| TEXAS INSTRUMENTS INCORPORATED
| Standard Linear and Logic Group
| IBIS Model of SN74LVC1G17
| SINGLE SCHMITT-TRIGGER BUFFER
| This file contains package information for the following:
|  SON 6-pin (DSF) package as [Component] LVC1G17_DSF
|  SOT 5-pin (DCK) package as [Component] LVC1G17_DCK
|  SOT 5-pin (DBV) package as [Component] LVC1G17_DBV
|  NanoStar WCSP 5-pin (YEA) package as [Component] LVC1G17_YEA
|  NanoFree WCSP 5-pin (YZA) package as [Component] LVC1G17_YZA
|  NanoStar WCSP 5-pin (YEP) package as [Component] LVC1G17_YEP
|  NanoFree WCSP 5-pin (YZP) package as [Component] LVC1G17_YZP
|  DSBGA 4-pin (YZV) package as [Component] LVC1G17_YZV
| This device can be powered at the following Vccs:
|  1.8 volt Vcc
|  2.5 volt Vcc
|  3.3 volt Vcc
|  5 volt Vcc
| This file provides unique models under the [Model Selector] for each Vcc.
| For operation at a specific Vcc, select the appropriate model after each
| [Model Selector] keyword.
[IBIS Ver]   3.2
[Comment char]  |_char
[File Name]   sn74lvc1g17.ibs
[File Rev]   1.4 | d_die
[Date]   03/06/2014
[Source]
| Texas Instruments Incorporated.
| Analog-eLab Design Center, HPA
| 12500 TI Blvd
| Dallas, TX -75243
[Notes]   Revision History:
| The following is an IBIS list for the LVC1G17.
| Please contact sllibis@ti.com with questions and
| comments concerning SLL IBIS models.
| - FILE REV HISTORY
| - 1.3 YZV package added on 12/21/05
| - Due to the fact that the Device is 5.5-V Input tolarent,
|   the pulldown model has some Non-Monotonic Warnings.
| - Power clamp data deleted as there is no power-clamp diode.
| - 1.4 DSF package added 03/06/2014.
[Disclaimer]
| Property of Texas Instruments Incorporated.  Unauthorized
| reproduction and/or distribution is strictly prohibited.
| This product is protected under copyright law.
| Created  2002, (C) Copyright  2002, Texas Instruments
| Incorporated, All Rights Reserved
| UNLESS THERE IS A SIGNED, WRITTEN AGREEMENT TO THE
| CONTRARY, TEXAS INSTRUMENTS (TI) IS PROVIDING THE IBIS
| MODELS  AND WITHOUT ANY WARRANTY, EXPRESSED OR
| IMPLIED.  TI assumes no liability for:
|  1) the accuracy of the IBIS models provided to your
|   company;
|  2) the proper functioning of these IBIS Models in your
|   design or for any resulting applications; or
|  3) infringement of patents, copyrights or intellectual
|   property rights resulting from your use of these IBIS
|   models.
| TI provides IBIS Models as a service to our customers.
| You and your company shall not distribute, sell or give
| these models to anyone else without prior written
| permission from TI.
| TI reserves the right to make changes to our products or
| to discontinue any semiconductor product or service
| without notice, and advises our customers to obtain the
| latest version of relevant information to verify, before
| placing orders, that the information being relied on is
| current.
| Please be aware that your receipt and use of the IBIS
| information provided shall serve as acceptance of these
| terms and conditions.  If you do not accept these terms,
| you should return or destroy the IBIS models and any
| other accompanying information immediately.
[Copyright]
(C) Copyright 2014 Texas Instruments Incorporated.All rights reserved.
| Component LVC1G17_DSF 6-pin SON
[Component]   LVC1G17_DSF
[Manufacturer]   Texas Instruments, Inc.
[Package]
|   typ   min   max
R_pkg   0.041145   0.03325   0.04904
L_pkg   0.422435nH  0.33414nH   0.51073nH
C_pkg   0.109645pF  0.10407pF   0.11522pF
[Pin]   signal_name   model_name   R_pin   L_pin   C_pin
1   nc   nc   0.00109   0.02796nH   0.07413pF
2   A   LVC1G17_IN   0.03325   0.33414nH   0.10407pF
3   GND   GND   0.04429   0.45885nH   0.11133pF
4   Y   LVC1G17_OUT   0.04904   0.51073nH   0.11522pF
5   nc   nc   0.00037   0.03788nH   0.07652pF
6   VCC   POWER   0.04377   0.44894nH   0.11085pF
| Component LVC1G17_DCK 5-pin SOT
[Component]   LVC1G17_DCK
[Manufacturer]   Texas Instruments, Inc.
[Package]
|   typ   min   max
R_pkg   2.000e-02   1.700e-02   2.500e-02
L_pkg   9.980e-10   8.810e-10   1.069e-09
C_pkg   1.460e-13   1.180e-13   2.050e-13
[Pin]   signal_name   model_name   R_pin   L_pin   C_pin
1   nc   nc   1.900e-02   1.069e-09   1.620e-13
2   A   LVC1G17_IN   1.800e-02   8.810e-10   1.210e-13
3   GND   GND   1.700e-02   1.031e-09   2.050e-13
4   Y   LVC1G17_OUT   2.000e-02   9.600e-10   1.240e-13
5   VCC   POWER   2.500e-02   1.049e-09   1.180e-13
| Component LVC1G17_DBV 5-pin SOT
[Component]   LVC1G17_DBV
[Manufacturer]   Texas Instruments, Inc.
[Package]
|   typ   min   max
R_pkg   2.500e-02   2.100e-02   2.900e-02
L_pkg   1.529e-09   1.312e-09   1.906e-09
C_pkg   1.560e-13   1.100e-13   2.400e-13
[Pin]   signal_name   model_name   R_pin   L_pin   C_pin
1   nc   nc   2.100e-02   1.511e-09   1.440e-13
2   A   LVC1G17_IN   2.300e-02   1.312e-09   1.380e-13
3   GND   GND   2.900e-02   1.906e-09   2.400e-13
4   Y   LVC1G17_OUT   2.600e-02   1.541e-09   1.500e-13
5   VCC   POWER   2.500e-02   1.374e-09   1.100e-13
| Component LVC1G17_YEA 5-pin NanoStar WCSP
[Component]   LVC1G17_YEA
[Manufacturer]   Texas Instruments, Inc.
[Package]
|   typ   min   max
R_pkg   0.001   0.001   0.001
L_pkg   0.021nH   0.021nH   0.021nH
C_pkg   0.046pF   0.045pF   0.047pF
[Pin]   signal_name   model_name   R_pin   L_pin   C_pin
1   DNU   nc   0.001   0.021nH   0.046pF
2   A   LVC1G17_IN   0.001   0.021nH   0.047pF
3   GND   GND   0.001   0.021nH   0.046pF
4   Y   LVC1G17_OUT   0.001   0.021nH   0.045pF
5   VCC   POWER   0.001   0.021nH   0.045pF
| Component LVC1G17_YZA 5-pin NanoFree WCSP
[Component]   LVC1G17_YZA
[Manufacturer]   Texas Instruments, Inc.
[Package]
|   typ   min   max
R_pkg   0.001   0.001   0.001
L_pkg   0.021nH   0.021nH   0.021nH
C_pkg   0.046pF   0.045pF   0.047pF
[Pin]   signal_name   model_name   R_pin   L_pin   C_pin
1   DNU   nc   0.001   0.021nH   0.046pF
2   A   LVC1G17_IN   0.001   0.021nH   0.047pF
3   GND   GND   0.001   0.021nH   0.046pF
4   Y   LVC1G17_OUT   0.001   0.021nH   0.045pF
5   VCC   POWER   0.001   0.021nH   0.045pF
| Component LVC1G17_YEP 5-pin NanoStar WCSP
[Component]   LVC1G17_YEP
[Manufacturer]   Texas Instruments, Inc.
[Package]
|   typ   min   max
R_pkg   0.001   0.001   0.001
L_pkg   0.021nH   0.021nH   0.021nH
C_pkg   0.046pF   0.045pF   0.047pF
[Pin]   signal_name   model_name   R_pin   L_pin   C_pin
1   DNU   nc   0.001   0.021nH   0.046pF
2   A   LVC1G17_IN   0.001   0.021nH   0.047pF
3   GND   GND   0.001   0.021nH   0.046pF
4   Y   LVC1G17_OUT   0.001   0.021nH   0.045pF
5   VCC   POWER   0.001   0.021nH   0.045pF
| Component LVC1G17_YZP 5-pin NanoFree WCSP
[Component]   LVC1G17_YZP
[Manufacturer]   Texas Instruments, Inc.
[Package]
|   typ   min   max
R_pkg   0.001   0.001   0.001
L_pkg   0.021nH   0.021nH   0.021nH
C_pkg   0.046pF   0.045pF   0.047pF
[Pin]   signal_name   model_name   R_pin   L_pin   C_pin
1   DNU   nc   0.001   0.021nH   0.046pF
2   A   LVC1G17_IN   0.001   0.021nH   0.047pF
3   GND   GND   0.001   0.021nH   0.046pF
4   Y   LVC1G17_OUT   0.001   0.021nH   0.045pF
5   VCC   POWER   0.001   0.021nH   0.045pF
| Component LVC1G17_YZV 4-pin DSBGA
[Component]   LVC1G17_YZV
[Manufacturer]   Texas Instruments, Inc.
[Package]
|   typ   min   max
R_pkg   1.000e-03   1.000e-03   1.000e-03
L_pkg   2.600e-11   2.600e-11   2.600e-11
C_pkg   1.400e-14   1.400e-14   1.400e-14
[Pin]   signal_name   model_name   R_pin   L_pin   C_pin
1   GND   GND   1.000e-03   2.600e-11   1.400e-14
2   A   LVC1G17_IN   1.000e-03   2.600e-11   1.400e-14
3   Y   LVC1G17_OUT   1.000e-03   2.600e-11   1.400e-14
4   VCC   POWER   1.000e-03   2.600e-11   1.400e-14
| Model LVC1G17_IN
[Model Selector]   LVC1G17_IN
LVC1G17_IN_18   1.8 volt Vcc
LVC1G17_IN_25   2.5 volt Vcc
LVC1G17_IN_33   3.3 volt Vcc
LVC1G17_IN_50   5 volt Vcc
| Model LVC1G17_OUT
[Model Selector]   LVC1G17_OUT
LVC1G17_OUT_18   1.8 volt Vcc
LVC1G17_OUT_25   2.5 volt Vcc
LVC1G17_OUT_33   3.3 volt Vcc
LVC1G17_OUT_50   5 volt Vcc
| Models and submodels in the file (8): LVC1G17_IN_18 (Input), LVC1G17_IN_25 (Input), LVC1G17_IN_33 (Input), LVC1G17_IN_50 (Input), LVC1G17_OUT_18 (Output), LVC1G17_OUT_25 (Output), LVC1G17_OUT_33 (Output), LVC1G17_OUT_50 (Output)
